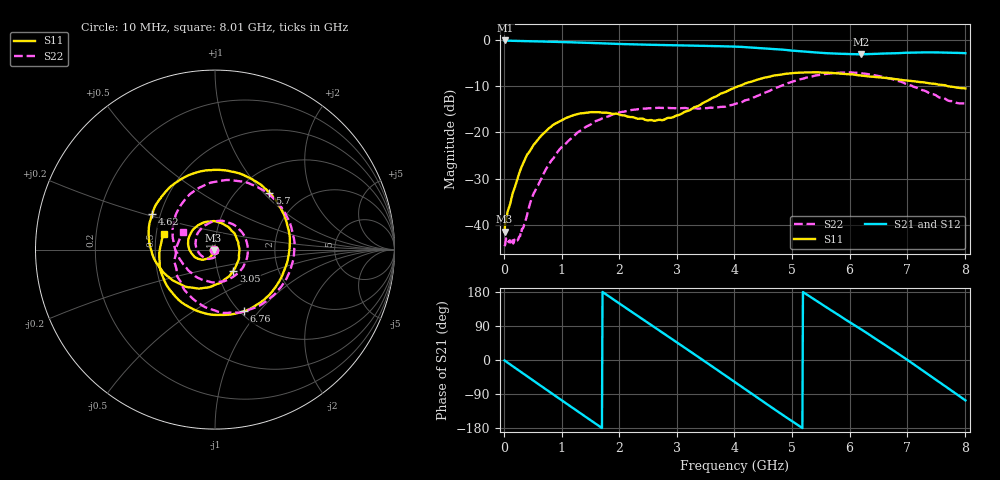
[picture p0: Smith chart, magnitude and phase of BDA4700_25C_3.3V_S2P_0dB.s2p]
!Agilent Technologies,E5071B,MY42404982,A.09.10
!Date: Mon Oct 20 18:02:58 2025
!Data & Calibration Information:
!Freq	S11:SOLT2(ON)	S21:SOLT2(ON)	S12:SOLT2(ON)	S22:SOLT2(ON)
# Hz S RI R 50
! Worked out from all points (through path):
!   801 points, 10 MHz to 8.01 GHz, reference 50 ohm
!   highest |S21| = -0.12 dB at 20 MHz (marker M1); lowest = -3.1 dB at 6.2 GHz (marker M2)
!   group delay of S21, straight-line fit = 285 ps
!   lowest |S11| = -41.5 dB at 10 MHz (marker M3), VSWR 1.02, Z = 49.2 - j0.254 ohm
!   |S11| at or under -10 dB: start of sweep to 4.071 GHz; 7.701 GHz to end of sweep
!   |S22| runs from -44.6 to -7.0 dB; largest |S21 - S12| = 0.011
!   S11 on the Smith chart (normalised r, x): 10 MHz: 0.98, -0.01; 3.05 GHz: 1.19, -0.29; 4.62 GHz: 0.45, +0.21; 5.7 GHz: 1.37, +1.08; 6.76 GHz: 1.04, -0.84; 8.01 GHz: 0.55, +0.11
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1e7  -0.00804 -0.00258  0.9855 -0.021  0.9852 -0.0219  -0.00588 -0.000379
2e7  -0.00935 -0.00458  0.985 -0.0384  0.9845 -0.0416  -0.00598 0.0014
3.4e8  -0.0259 -0.0401  0.7798 -0.5769  0.78 -0.5772  0.00946 0.00153
7.2e8  -0.0876 -0.0532  0.2207 -0.9322  0.2215 -0.932  0.00194 -0.0393
1.02e9  -0.1367 -0.0116  -0.2963 -0.8994  -0.2966 -0.8997  -0.0519 -0.0482
1.35e9  -0.1443 0.0703  -0.7451 -0.5625  -0.745 -0.563  -0.1056 0.0152
1.92e9  -0.016 0.1582  -0.8391 0.345  -0.8398 0.3448  0.00104 0.1583
2.32e9  0.0934 0.1044  -0.3981 0.7977  -0.3979 0.7975  0.1465 0.1009
2.68e9  0.1363 0.0018  0.1603 0.867  0.1592 0.8669  0.1779 -0.0486
3.05e9  0.1014 -0.1174  0.6563 0.5756  0.6507 0.58  0.0808 -0.1635
3.52e9  -0.0497 -0.2118  0.8544 -0.1083  0.8553 -0.1095  -0.0883 -0.1601
4.01e9  -0.2681 -0.1459  0.4411 -0.7203  0.4427 -0.719  -0.1952 -0.0532
4.62e9  -0.3498 0.1964  -0.4296 -0.6773  -0.4283 -0.6779  -0.2242 0.1731
4.99e9  -0.1899 0.3921  -0.7223 -0.2576  -0.7237 -0.2598  -0.1025 0.3356
5.35e9  0.0688 0.4396  -0.706 0.2113  -0.7074 0.2073  0.1264 0.3823
5.7e9  0.3021 0.3174  -0.4497 0.5538  -0.4492 0.554  0.3485 0.2626
6.2e9  0.4099 -0.0342  0.1108 0.69  0.1206 0.6918  0.4231 -0.1015
6.68e9  0.2133 -0.3201  0.5971 0.3886  0.5994 0.3886  0.1796 -0.3382
6.76e9  0.161 -0.3439  0.6479 0.3044  0.651 0.2999  0.1268 -0.3515
7.29e9  -0.1901 -0.2905  0.6344 -0.3669  0.6343 -0.3673  -0.1663 -0.2295
7.66e9  -0.3078 -0.0958  0.2581 -0.6804  0.2577 -0.6812  -0.2254 -0.0531
8.01e9  -0.285 0.0886  -0.205 -0.6882  -0.2024 -0.6895  -0.1791 0.0991
